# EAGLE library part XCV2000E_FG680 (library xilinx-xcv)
xcv2000e_fg680 edit this description Auto generated by make-symbol-device-package-bsdl.ulp Rev. 26 Source: xcv2000e_fg680.bsd
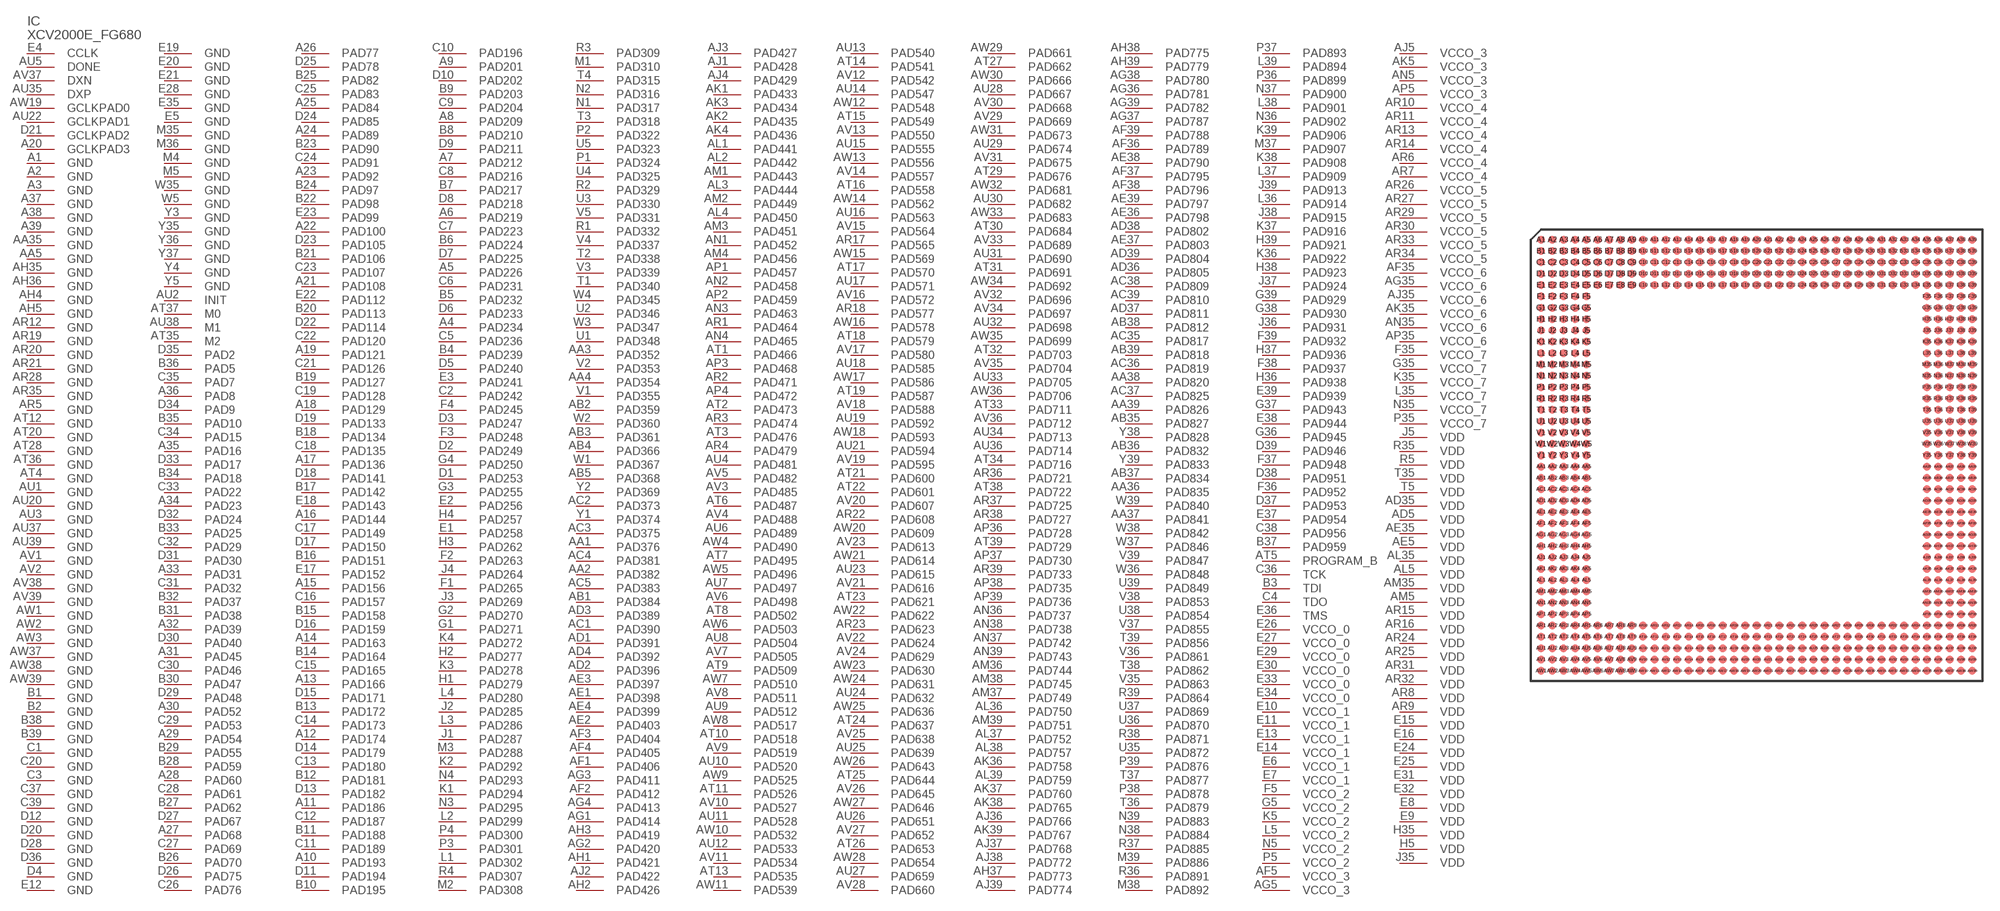
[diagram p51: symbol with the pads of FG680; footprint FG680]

Designator prefix IC

## XCV2000E_FG680 (OC_FARNELL: unknown; OC_NEWARK: unknown)  [FG680]
A1  GND  pwr
A2  GND  pwr
A3  GND  pwr
A4  PAD234
A5  PAD226
A6  PAD219
A7  PAD212
A8  PAD209
A9  PAD201
A10  PAD193
A11  PAD186
A12  PAD174
A13  PAD166
A14  PAD163
A15  PAD156
A16  PAD144
A17  PAD136
A18  PAD129
A19  PAD121
A20  GCLKPAD3  in
A21  PAD108
A22  PAD100
A23  PAD92
A24  PAD89
A25  PAD84
A26  PAD77
A27  PAD68
A28  PAD60
A29  PAD54
A30  PAD52
A31  PAD45
A32  PAD39
A33  PAD31
A34  PAD23
A35  PAD16
A36  PAD8
A37  GND  pwr
A38  GND  pwr
A39  GND  pwr
AA1  PAD376
AA2  PAD382
AA3  PAD352
AA4  PAD354
AA5  GND  pwr
AA35  GND  pwr
AA36  PAD835
AA37  PAD841
AA38  PAD820
AA39  PAD826
AB1  PAD384
AB2  PAD359
AB3  PAD361
AB4  PAD366
AB5  PAD368
AB35  PAD827
AB36  PAD832
AB37  PAD834
AB38  PAD812
AB39  PAD818
AC1  PAD390
AC2  PAD373
AC3  PAD375
AC4  PAD381
AC5  PAD383
AC35  PAD817
AC36  PAD819
AC37  PAD825
AC38  PAD809
AC39  PAD810
AD1  PAD391
AD2  PAD396
AD3  PAD389
AD4  PAD392
AD5  VDD  pwr
AD35  VDD  pwr
AD36  PAD805
AD37  PAD811
AD38  PAD802
AD39  PAD804
AE1  PAD398
AE2  PAD403
AE3  PAD397
AE4  PAD399
AE5  VDD  pwr
AE35  VDD  pwr
AE36  PAD798
AE37  PAD803
AE38  PAD790
AE39  PAD797
AF1  PAD406
AF2  PAD412
AF3  PAD404
AF4  PAD405
AF5  VCCO_3  pwr
AF35  VCCO_6  pwr
AF36  PAD789
AF37  PAD795
AF38  PAD796
AF39  PAD788
AG1  PAD414
AG2  PAD420
AG3  PAD411
AG4  PAD413
AG5  VCCO_3  pwr
AG35  VCCO_6  pwr
AG36  PAD781
AG37  PAD787
AG38  PAD780
AG39  PAD782
AH1  PAD421
AH2  PAD426
AH3  PAD419
AH4  GND  pwr
AH5  GND  pwr
AH35  GND  pwr
AH36  GND  pwr
AH37  PAD773
AH38  PAD775
AH39  PAD779
AJ1  PAD428
AJ2  PAD422
AJ3  PAD427
AJ4  PAD429
AJ5  VCCO_3  pwr
AJ35  VCCO_6  pwr
AJ36  PAD766
AJ37  PAD768
AJ38  PAD772
AJ39  PAD774
AK1  PAD433
AK2  PAD435
AK3  PAD434
AK4  PAD436
AK5  VCCO_3  pwr
AK35  VCCO_6  pwr
AK36  PAD758
AK37  PAD760
AK38  PAD765
AK39  PAD767
AL1  PAD441
AL2  PAD442
AL3  PAD444
AL4  PAD450
AL5  VDD  pwr
AL35  VDD  pwr
AL36  PAD750
AL37  PAD752
AL38  PAD757
AL39  PAD759
AM1  PAD443
AM2  PAD449
AM3  PAD451
AM4  PAD456
AM5  VDD  pwr
AM35  VDD  pwr
AM36  PAD744
AM37  PAD749
AM38  PAD745
AM39  PAD751
AN1  PAD452
AN2  PAD458
AN3  PAD463
AN4  PAD465
AN5  VCCO_3  pwr
AN35  VCCO_6  pwr
AN36  PAD737
AN37  PAD742
AN38  PAD738
AN39  PAD743
AP1  PAD457
AP2  PAD459
AP3  PAD468
AP4  PAD472
AP5  VCCO_3  pwr
AP35  VCCO_6  pwr
AP36  PAD728
AP37  PAD730
AP38  PAD735
AP39  PAD736
AR1  PAD464
AR2  PAD471
AR3  PAD474
AR4  PAD479
AR5  GND  pwr
AR6  VCCO_4  pwr
AR7  VCCO_4  pwr
AR8  VDD  pwr
AR9  VDD  pwr
AR10  VCCO_4  pwr
AR11  VCCO_4  pwr
AR12  GND  pwr
AR13  VCCO_4  pwr
AR14  VCCO_4  pwr
AR15  VDD  pwr
AR16  VDD  pwr
AR17  PAD565
AR18  PAD577
AR19  GND  pwr
AR20  GND  pwr
AR21  GND  pwr
AR22  PAD608
AR23  PAD623
AR24  VDD  pwr
AR25  VDD  pwr
AR26  VCCO_5  pwr
AR27  VCCO_5  pwr
AR28  GND  pwr
AR29  VCCO_5  pwr
AR30  VCCO_5  pwr
AR31  VDD  pwr
AR32  VDD  pwr
AR33  VCCO_5  pwr
AR34  VCCO_5  pwr
AR35  GND  pwr
AR36  PAD721
AR37  PAD725
AR38  PAD727
AR39  PAD733
AT1  PAD466
AT2  PAD473
AT3  PAD476
AT4  GND  pwr
AT5  PROGRAM_B  in
AT6  PAD487
AT7  PAD495
AT8  PAD502
AT9  PAD509
AT10  PAD518
AT11  PAD526
AT12  GND  pwr
AT13  PAD535
AT14  PAD541
AT15  PAD549
AT16  PAD558
AT17  PAD570
AT18  PAD579
AT19  PAD587
AT20  GND  pwr
AT21  PAD600
AT22  PAD601
AT23  PAD621
AT24  PAD637
AT25  PAD644
AT26  PAD653
AT27  PAD662
AT28  GND  pwr
AT29  PAD676
AT30  PAD684
AT31  PAD691
AT32  PAD703
AT33  PAD711
AT34  PAD716
AT35  M2  in
AT36  GND  pwr
AT37  M0  in
AT38  PAD722
AT39  PAD729
AU1  GND  pwr
AU2  INIT
AU3  GND  pwr
AU4  PAD481
AU5  DONE
AU6  PAD489
AU7  PAD497
AU8  PAD504
AU9  PAD512
AU10  PAD520
AU11  PAD528
AU12  PAD533
AU13  PAD540
AU14  PAD547
AU15  PAD555
AU16  PAD563
AU17  PAD571
AU18  PAD585
AU19  PAD592
AU20  GND  pwr
AU21  PAD594
AU22  GCLKPAD1  in
AU23  PAD615
AU24  PAD632
AU25  PAD639
AU26  PAD651
AU27  PAD659
AU28  PAD667
AU29  PAD674
AU30  PAD682
AU31  PAD690
AU32  PAD698
AU33  PAD705
AU34  PAD713
AU35  DXP  pas
AU36  PAD714
AU37  GND  pwr
AU38  M1  in
AU39  GND  pwr
AV1  GND  pwr
AV2  GND  pwr
AV3  PAD485
AV4  PAD488
AV5  PAD482
AV6  PAD498
AV7  PAD505
AV8  PAD511
AV9  PAD519
AV10  PAD527
AV11  PAD534
AV12  PAD542
AV13  PAD550
AV14  PAD557
AV15  PAD564
AV16  PAD572
AV17  PAD580
AV18  PAD588
AV19  PAD595
AV20  PAD607
AV21  PAD616
AV22  PAD624
AV23  PAD613
AV24  PAD629
AV25  PAD638
AV26  PAD645
AV27  PAD652
AV28  PAD660
AV29  PAD669
AV30  PAD668
AV31  PAD675
AV32  PAD696
AV33  PAD689
AV34  PAD697
AV35  PAD704
AV36  PAD712
AV37  DXN  pas
AV38  GND  pwr
AV39  GND  pwr
AW1  GND  pwr
AW2  GND  pwr
AW3  GND  pwr
AW4  PAD490
AW5  PAD496
AW6  PAD503
AW7  PAD510
AW8  PAD517
AW9  PAD525
AW10  PAD532
AW11  PAD539
AW12  PAD548
AW13  PAD556
AW14  PAD562
AW15  PAD569
AW16  PAD578
AW17  PAD586
AW18  PAD593
AW19  GCLKPAD0  in
AW20  PAD609
AW21  PAD614
AW22  PAD622
AW23  PAD630
AW24  PAD631
AW25  PAD636
AW26  PAD643
AW27  PAD646
AW28  PAD654
AW29  PAD661
AW30  PAD666
AW31  PAD673
AW32  PAD681
AW33  PAD683
AW34  PAD692
AW35  PAD699
AW36  PAD706
AW37  GND  pwr
AW38  GND  pwr
AW39  GND  pwr
B1  GND  pwr
B2  GND  pwr
B3  TDI  in
B4  PAD239
B5  PAD232
B6  PAD224
B7  PAD217
B8  PAD210
B9  PAD203
B10  PAD195
B11  PAD188
B12  PAD181
B13  PAD172
B14  PAD164
B15  PAD158
B16  PAD151
B17  PAD142
B18  PAD134
B19  PAD127
B20  PAD113
B21  PAD106
B22  PAD98
B23  PAD90
B24  PAD97
B25  PAD82
B26  PAD70
B27  PAD62
B28  PAD59
B29  PAD55
B30  PAD47
B31  PAD38
B32  PAD37
B33  PAD25
B34  PAD18
B35  PAD10
B36  PAD5
B37  PAD959
B38  GND  pwr
B39  GND  pwr
C1  GND  pwr
C2  PAD242
C3  GND  pwr
C4  TDO  out
C5  PAD236
C6  PAD231
C7  PAD223
C8  PAD216
C9  PAD204
C10  PAD196
C11  PAD189
C12  PAD187
C13  PAD180
C14  PAD173
C15  PAD165
C16  PAD157
C17  PAD149
C18  PAD135
C19  PAD128
C20  GND  pwr
C21  PAD126
C22  PAD120
C23  PAD107
C24  PAD91
C25  PAD83
C26  PAD76
C27  PAD69
C28  PAD61
C29  PAD53
C30  PAD46
C31  PAD32
C32  PAD29
C33  PAD22
C34  PAD15
C35  PAD7
C36  TCK  in
C37  GND  pwr
C38  PAD956
C39  GND  pwr
D1  PAD253
D2  PAD249
D3  PAD247
D4  GND  pwr
D5  PAD240
D6  PAD233
D7  PAD225
D8  PAD218
D9  PAD211
D10  PAD202
D11  PAD194
D12  GND  pwr
D13  PAD182
D14  PAD179
D15  PAD171
D16  PAD159
D17  PAD150
D18  PAD141
D19  PAD133
D20  GND  pwr
D21  GCLKPAD2  in
D22  PAD114
D23  PAD105
D24  PAD85
D25  PAD78
D26  PAD75
D27  PAD67
D28  GND  pwr
D29  PAD48
D30  PAD40
D31  PAD30
D32  PAD24
D33  PAD17
D34  PAD9
D35  PAD2
D36  GND  pwr
D37  PAD953
D38  PAD951
D39  PAD946
E1  PAD258
E2  PAD256
E3  PAD241
E4  CCLK
E5  GND  pwr
E6  VCCO_1  pwr
E7  VCCO_1  pwr
E8  VDD  pwr
E9  VDD  pwr
E10  VCCO_1  pwr
E11  VCCO_1  pwr
E12  GND  pwr
E13  VCCO_1  pwr
E14  VCCO_1  pwr
E15  VDD  pwr
E16  VDD  pwr
E17  PAD152
E18  PAD143
E19  GND  pwr
E20  GND  pwr
E21  GND  pwr
E22  PAD112
E23  PAD99
E24  VDD  pwr
E25  VDD  pwr
E26  VCCO_0  pwr
E27  VCCO_0  pwr
E28  GND  pwr
E29  VCCO_0  pwr
E30  VCCO_0  pwr
E31  VDD  pwr
E32  VDD  pwr
E33  VCCO_0  pwr
E34  VCCO_0  pwr
E35  GND  pwr
E36  TMS  in
E37  PAD954
E38  PAD944
E39  PAD939
F1  PAD265
F2  PAD263
F3  PAD248
F4  PAD245
F5  VCCO_2  pwr
F35  VCCO_7  pwr
F36  PAD952
F37  PAD948
F38  PAD937
F39  PAD932
G1  PAD271
G2  PAD270
G3  PAD255
G4  PAD250
G5  VCCO_2  pwr
G35  VCCO_7  pwr
G36  PAD945
G37  PAD943
G38  PAD930
G39  PAD929
H1  PAD279
H2  PAD277
H3  PAD262
H4  PAD257
H5  VDD  pwr
H35  VDD  pwr
H36  PAD938
H37  PAD936
H38  PAD923
H39  PAD921
J1  PAD287
J2  PAD285
J3  PAD269
J4  PAD264
J5  VDD  pwr
J35  VDD  pwr
J36  PAD931
J37  PAD924
J38  PAD915
J39  PAD913
K1  PAD294
K2  PAD292
K3  PAD278
K4  PAD272
K5  VCCO_2  pwr
K35  VCCO_7  pwr
K36  PAD922
K37  PAD916
K38  PAD908
K39  PAD906
L1  PAD302
L2  PAD299
L3  PAD286
L4  PAD280
L5  VCCO_2  pwr
L35  VCCO_7  pwr
L36  PAD914
L37  PAD909
L38  PAD901
L39  PAD894
M1  PAD310
M2  PAD308
M3  PAD288
M4  GND  pwr
M5  GND  pwr
M35  GND  pwr
M36  GND  pwr
M37  PAD907
M38  PAD892
M39  PAD886
N1  PAD317
N2  PAD316
N3  PAD295
N4  PAD293
N5  VCCO_2  pwr
N35  VCCO_7  pwr
N36  PAD902
N37  PAD900
N38  PAD884
N39  PAD883
P1  PAD324
P2  PAD322
P3  PAD301
P4  PAD300
P5  VCCO_2  pwr
P35  VCCO_7  pwr
P36  PAD899
P37  PAD893
P38  PAD878
P39  PAD876
R1  PAD332
R2  PAD329
R3  PAD309
R4  PAD307
R5  VDD  pwr
R35  VDD  pwr
R36  PAD891
R37  PAD885
R38  PAD871
R39  PAD864
T1  PAD340
T2  PAD338
T3  PAD318
T4  PAD315
T5  VDD  pwr
T35  VDD  pwr
T36  PAD879
T37  PAD877
T38  PAD862
T39  PAD856
U1  PAD348
U2  PAD346
U3  PAD330
U4  PAD325
U5  PAD323
U35  PAD872
U36  PAD870
U37  PAD869
U38  PAD854
U39  PAD849
V1  PAD355
V2  PAD353
V3  PAD339
V4  PAD337
V5  PAD331
V35  PAD863
V36  PAD861
V37  PAD855
V38  PAD853
V39  PAD847
W1  PAD367
W2  PAD360
W3  PAD347
W4  PAD345
W5  GND  pwr
W35  GND  pwr
W36  PAD848
W37  PAD846
W38  PAD842
W39  PAD840
Y1  PAD374
Y2  PAD369
Y3  GND  pwr
Y4  GND  pwr
Y5  GND  pwr
Y35  GND  pwr
Y36  GND  pwr
Y37  GND  pwr
Y38  PAD828
Y39  PAD833

## Footprint FG680 (pad centres in mm)
xcv1000_fg680_1532 edit this description Auto generated by make-symbol-device-package-bsdl.ulp Rev. 26 Source: xcv1000_fg680_1532.bsd
smd 0.7 x 0.7: A1 -19,19; A2 -18,19; A3 -17,19; A4 -16,19; A5 -15,19; A6 -14,19; A7 -13,19; A8 -12,19; A9 -11,19; A10 -10,19; A11 -9,19; A12 -8,19; A13 -7,19; A14 -6,19; A15 -5,19; A16 -4,19; A17 -3,19; A18 -2,19; A19 -1,19; A20 0,19; A21 1,19; A22 2,19; A23 3,19; A24 4,19; A25 5,19; A26 6,19; A27 7,19; A28 8,19; A29 9,19; A30 10,19; A31 11,19; A32 12,19; A33 13,19; A34 14,19; A35 15,19; A36 16,19; A37 17,19; A38 18,19; A39 19,19; AA1 -19,-1; AA2 -18,-1; AA3 -17,-1; AA4 -16,-1; AA5 -15,-1; AA35 15,-1; AA36 16,-1; AA37 17,-1; AA38 18,-1; AA39 19,-1; AB1 -19,-2; AB2 -18,-2; AB3 -17,-2; AB4 -16,-2; AB5 -15,-2; AB35 15,-2; AB36 16,-2; AB37 17,-2; AB38 18,-2; AB39 19,-2; AC1 -19,-3; AC2 -18,-3; AC3 -17,-3; AC4 -16,-3; AC5 -15,-3; AC35 15,-3; AC36 16,-3; AC37 17,-3; AC38 18,-3; AC39 19,-3; AD1 -19,-4; AD2 -18,-4; AD3 -17,-4; AD4 -16,-4; AD5 -15,-4; AD35 15,-4; AD36 16,-4; AD37 17,-4; AD38 18,-4; AD39 19,-4; AE1 -19,-5; AE2 -18,-5; AE3 -17,-5; AE4 -16,-5; AE5 -15,-5; AE35 15,-5; AE36 16,-5; AE37 17,-5; AE38 18,-5; AE39 19,-5; AF1 -19,-6; AF2 -18,-6; AF3 -17,-6; AF4 -16,-6; AF5 -15,-6; AF35 15,-6; AF36 16,-6; AF37 17,-6; AF38 18,-6; AF39 19,-6; AG1 -19,-7; AG2 -18,-7; AG3 -17,-7; AG4 -16,-7; AG5 -15,-7; AG35 15,-7; AG36 16,-7; AG37 17,-7; AG38 18,-7; AG39 19,-7; AH1 -19,-8; AH2 -18,-8; AH3 -17,-8; AH4 -16,-8; AH5 -15,-8; AH35 15,-8; AH36 16,-8; AH37 17,-8; AH38 18,-8; AH39 19,-8; AJ1 -19,-9; AJ2 -18,-9; AJ3 -17,-9; AJ4 -16,-9; AJ5 -15,-9; AJ35 15,-9; AJ36 16,-9; AJ37 17,-9; AJ38 18,-9; AJ39 19,-9; AK1 -19,-10; AK2 -18,-10; AK3 -17,-10; AK4 -16,-10; AK5 -15,-10; AK35 15,-10; AK36 16,-10; AK37 17,-10; AK38 18,-10; AK39 19,-10; AL1 -19,-11; AL2 -18,-11; AL3 -17,-11; AL4 -16,-11; AL5 -15,-11; AL35 15,-11; AL36 16,-11; AL37 17,-11; AL38 18,-11; AL39 19,-11; AM1 -19,-12; AM2 -18,-12; AM3 -17,-12; AM4 -16,-12; AM5 -15,-12; AM35 15,-12; AM36 16,-12; AM37 17,-12; AM38 18,-12; AM39 19,-12; AN1 -19,-13; AN2 -18,-13; AN3 -17,-13; AN4 -16,-13; AN5 -15,-13; AN35 15,-13; AN36 16,-13; AN37 17,-13; AN38 18,-13; AN39 19,-13; AP1 -19,-14; AP2 -18,-14; AP3 -17,-14; AP4 -16,-14; AP5 -15,-14; AP35 15,-14; AP36 16,-14; AP37 17,-14; AP38 18,-14; AP39 19,-14; AR1 -19,-15; AR2 -18,-15; AR3 -17,-15; AR4 -16,-15; AR5 -15,-15; AR6 -14,-15; AR7 -13,-15; AR8 -12,-15; AR9 -11,-15; AR10 -10,-15; AR11 -9,-15; AR12 -8,-15; AR13 -7,-15; AR14 -6,-15; AR15 -5,-15; AR16 -4,-15; AR17 -3,-15; AR18 -2,-15; AR19 -1,-15; AR20 0,-15; AR21 1,-15; AR22 2,-15; AR23 3,-15; AR24 4,-15; AR25 5,-15; AR26 6,-15; AR27 7,-15; AR28 8,-15; AR29 9,-15; AR30 10,-15; AR31 11,-15; AR32 12,-15; AR33 13,-15; AR34 14,-15; AR35 15,-15; AR36 16,-15; AR37 17,-15; AR38 18,-15; AR39 19,-15; AT1 -19,-16; AT2 -18,-16; AT3 -17,-16; AT4 -16,-16; AT5 -15,-16; AT6 -14,-16; AT7 -13,-16; AT8 -12,-16; AT9 -11,-16; AT10 -10,-16; AT11 -9,-16; AT12 -8,-16; AT13 -7,-16; AT14 -6,-16; AT15 -5,-16; AT16 -4,-16; AT17 -3,-16; AT18 -2,-16; AT19 -1,-16; AT20 0,-16; AT21 1,-16; AT22 2,-16; AT23 3,-16; AT24 4,-16; AT25 5,-16; AT26 6,-16; AT27 7,-16; AT28 8,-16; AT29 9,-16; AT30 10,-16; AT31 11,-16; AT32 12,-16; AT33 13,-16; AT34 14,-16; AT35 15,-16; AT36 16,-16; AT37 17,-16; AT38 18,-16; AT39 19,-16; AU1 -19,-17; AU2 -18,-17; AU3 -17,-17; AU4 -16,-17; AU5 -15,-17; AU6 -14,-17; AU7 -13,-17; AU8 -12,-17; AU9 -11,-17; AU10 -10,-17; AU11 -9,-17; AU12 -8,-17; AU13 -7,-17; AU14 -6,-17; AU15 -5,-17; AU16 -4,-17; AU17 -3,-17; AU18 -2,-17; AU19 -1,-17; AU20 0,-17; AU21 1,-17; AU22 2,-17; AU23 3,-17; AU24 4,-17; AU25 5,-17; AU26 6,-17; AU27 7,-17; AU28 8,-17; AU29 9,-17; AU30 10,-17; AU31 11,-17; AU32 12,-17; AU33 13,-17; AU34 14,-17; AU35 15,-17; AU36 16,-17; AU37 17,-17; AU38 18,-17; AU39 19,-17; AV1 -19,-18; AV2 -18,-18; AV3 -17,-18; AV4 -16,-18; AV5 -15,-18; AV6 -14,-18; AV7 -13,-18; AV8 -12,-18; AV9 -11,-18; AV10 -10,-18; AV11 -9,-18; AV12 -8,-18; AV13 -7,-18; AV14 -6,-18; AV15 -5,-18; AV16 -4,-18; AV17 -3,-18; AV18 -2,-18; AV19 -1,-18; AV20 0,-18; AV21 1,-18; AV22 2,-18; AV23 3,-18; AV24 4,-18; AV25 5,-18; AV26 6,-18; AV27 7,-18; AV28 8,-18; AV29 9,-18; AV30 10,-18; AV31 11,-18; AV32 12,-18; AV33 13,-18; AV34 14,-18; AV35 15,-18; AV36 16,-18; AV37 17,-18; AV38 18,-18; AV39 19,-18; AW1 -19,-19; AW2 -18,-19; AW3 -17,-19; AW4 -16,-19; AW5 -15,-19; AW6 -14,-19; AW7 -13,-19; AW8 -12,-19; AW9 -11,-19; AW10 -10,-19; AW11 -9,-19; AW12 -8,-19; AW13 -7,-19; AW14 -6,-19; AW15 -5,-19; AW16 -4,-19; AW17 -3,-19; AW18 -2,-19; AW19 -1,-19; AW20 0,-19; AW21 1,-19; AW22 2,-19; AW23 3,-19; AW24 4,-19; AW25 5,-19; AW26 6,-19; AW27 7,-19; AW28 8,-19; AW29 9,-19; AW30 10,-19; AW31 11,-19; AW32 12,-19; AW33 13,-19; AW34 14,-19; AW35 15,-19; AW36 16,-19; AW37 17,-19; AW38 18,-19; AW39 19,-19; B1 -19,18; B2 -18,18; B3 -17,18; B4 -16,18; B5 -15,18; B6 -14,18; B7 -13,18; B8 -12,18; B9 -11,18; B10 -10,18; B11 -9,18; B12 -8,18; B13 -7,18; B14 -6,18; B15 -5,18; B16 -4,18; B17 -3,18; B18 -2,18; B19 -1,18; B20 0,18; B21 1,18; B22 2,18; B23 3,18; B24 4,18; B25 5,18; B26 6,18; B27 7,18; B28 8,18; B29 9,18; B30 10,18; B31 11,18; B32 12,18; B33 13,18; B34 14,18; B35 15,18; B36 16,18; B37 17,18; B38 18,18; B39 19,18; C1 -19,17; C2 -18,17; C3 -17,17; C4 -16,17; C5 -15,17; C6 -14,17; C7 -13,17; C8 -12,17; C9 -11,17; C10 -10,17; C11 -9,17; C12 -8,17; C13 -7,17; C14 -6,17; C15 -5,17; C16 -4,17; C17 -3,17; C18 -2,17; C19 -1,17; C20 0,17; C21 1,17; C22 2,17; C23 3,17; C24 4,17; C25 5,17; C26 6,17; C27 7,17; C28 8,17; C29 9,17; C30 10,17; C31 11,17; C32 12,17; C33 13,17; C34 14,17; C35 15,17; C36 16,17; C37 17,17; C38 18,17; C39 19,17; D1 -19,16; D2 -18,16; D3 -17,16; D4 -16,16; D5 -15,16; D6 -14,16; D7 -13,16; D8 -12,16; D9 -11,16; D10 -10,16; D11 -9,16; D12 -8,16; D13 -7,16; D14 -6,16; D15 -5,16; D16 -4,16; D17 -3,16; D18 -2,16; D19 -1,16; D20 0,16; D21 1,16; D22 2,16; D23 3,16; D24 4,16; D25 5,16; D26 6,16; D27 7,16; D28 8,16; D29 9,16; D30 10,16; D31 11,16; D32 12,16; D33 13,16; D34 14,16; D35 15,16; D36 16,16; D37 17,16; D38 18,16; D39 19,16; E1 -19,15; E2 -18,15; E3 -17,15; E4 -16,15; E5 -15,15; E6 -14,15; E7 -13,15; E8 -12,15; E9 -11,15; E10 -10,15; E11 -9,15; E12 -8,15; E13 -7,15; E14 -6,15; E15 -5,15; E16 -4,15; E17 -3,15; E18 -2,15; E19 -1,15; E20 0,15; E21 1,15; E22 2,15; E23 3,15; E24 4,15; E25 5,15; E26 6,15; E27 7,15; E28 8,15; E29 9,15; E30 10,15; E31 11,15; E32 12,15; E33 13,15; E34 14,15; E35 15,15; E36 16,15; E37 17,15; E38 18,15; E39 19,15; F1 -19,14; F2 -18,14; F3 -17,14; F4 -16,14; F5 -15,14; F35 15,14; F36 16,14; F37 17,14; F38 18,14; F39 19,14; G1 -19,13; G2 -18,13; G3 -17,13; G4 -16,13; G5 -15,13; G35 15,13; G36 16,13; G37 17,13; G38 18,13; G39 19,13; H1 -19,12; H2 -18,12; H3 -17,12; H4 -16,12; H5 -15,12; H35 15,12; H36 16,12; H37 17,12; H38 18,12; H39 19,12; J1 -19,11; J2 -18,11; J3 -17,11; J4 -16,11; J5 -15,11; J35 15,11; J36 16,11; J37 17,11; J38 18,11; J39 19,11; K1 -19,10; K2 -18,10; K3 -17,10; K4 -16,10; K5 -15,10; K35 15,10; K36 16,10; K37 17,10; K38 18,10; K39 19,10; L1 -19,9; L2 -18,9; L3 -17,9; L4 -16,9; L5 -15,9; L35 15,9; L36 16,9; L37 17,9; L38 18,9; L39 19,9; M1 -19,8; M2 -18,8; M3 -17,8; M4 -16,8; M5 -15,8; M35 15,8; M36 16,8; M37 17,8; M38 18,8; M39 19,8; N1 -19,7; N2 -18,7; N3 -17,7; N4 -16,7; N5 -15,7; N35 15,7; N36 16,7; N37 17,7; N38 18,7; N39 19,7; P1 -19,6; P2 -18,6; P3 -17,6; P4 -16,6; P5 -15,6; P35 15,6; P36 16,6; P37 17,6; P38 18,6; P39 19,6; R1 -19,5; R2 -18,5; R3 -17,5; R4 -16,5; R5 -15,5; R35 15,5; R36 16,5; R37 17,5; R38 18,5; R39 19,5; T1 -19,4; T2 -18,4; T3 -17,4; T4 -16,4; T5 -15,4; T35 15,4; T36 16,4; T37 17,4; T38 18,4; T39 19,4; U1 -19,3; U2 -18,3; U3 -17,3; U4 -16,3; U5 -15,3; U35 15,3; U36 16,3; U37 17,3; U38 18,3; U39 19,3; V1 -19,2; V2 -18,2; V3 -17,2; V4 -16,2; V5 -15,2; V35 15,2; V36 16,2; V37 17,2; V38 18,2; V39 19,2; W1 -19,1; W2 -18,1; W3 -17,1; W4 -16,1; W5 -15,1; W35 15,1; W36 16,1; W37 17,1; W38 18,1; W39 19,1; Y1 -19,0; Y2 -18,0; Y3 -17,0; Y4 -16,0; Y5 -15,0; Y35 15,0; Y36 16,0; Y37 17,0; Y38 18,0; Y39 19,0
